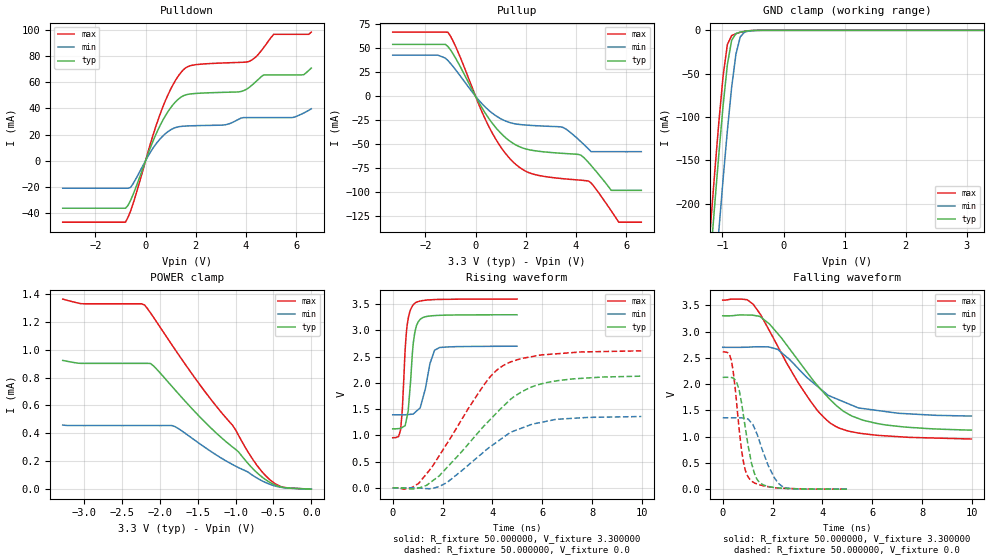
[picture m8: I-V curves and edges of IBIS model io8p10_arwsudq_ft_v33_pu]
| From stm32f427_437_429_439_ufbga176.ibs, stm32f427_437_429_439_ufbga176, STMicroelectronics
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|   Model io8p10_arwsudq_ft_v33_pu
[Model]  io8p10_arwsudq_ft_v33_pu
Model_type I/O
Polarity   Non-Inverting
Enable   Active-Low
Vinl =   0.990000V
Vinh =   2.310000V
Vmeas =  1.650000V
Cref =   40.000000pF
Rref =   100.000000M
Vref =   0.0V
C_comp   2.911600pF   2.823500pF   2.988000pF
[Temperature Range]   25.000000   0.125000k   -40.000000
[Pullup Reference]   3.300000V   2.700000V   3.600000V
[Pulldown Reference]   0.0V   0.0V   0.0V
[POWER Clamp Reference]   3.300000V   2.700000V   3.600000V
[GND Clamp Reference]   0.0V   0.0V   0.0V
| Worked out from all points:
|   slope of the pulldown table from 0 to 0.495 V, typ, clamps not added: 20.9 ohm
|   slope of the pullup table from 0 to 0.495 V, typ, clamps not added: 22.6 ohm
|   GND clamp passes 1 mA (typ) near -0.62 V on its own axis
|   rising waveform, R_fixture 50.000000, V_fixture 3.300000: 20-80 % time 219ps typ, 369ps min, 188ps max; typ from 1.12 V to 3.3 V
|   rising waveform, R_fixture 50.000000, V_fixture 0.0: 20-80 % time 2.52ns typ, 2.26ns min, 2.12ns max; typ from 0.001 V to 2.13 V
|   falling waveform, R_fixture 50.000000, V_fixture 3.300000: 20-80 % time 2.26ns typ, 2.15ns min, 2.01ns max; typ from 3.3 V to 1.12 V
|   falling waveform, R_fixture 50.000000, V_fixture 0.0: 20-80 % time 465ps typ, 673ps min, 372ps max; typ from 2.13 V to 0.001 V
[Pulldown]
|Voltage   I(typ)   I(min)   I(max)
-3.3V     -36.38mA   -21.07mA   -47.09mA
-800mV    -36.38mA   -21.07mA   -47.09mA
-600mV    -30.5mA    -20.54mA   -38.69mA
700mV     31.4mA     19.11mA    41.71mA
1.2V      45.15mA    25.37mA    61.75mA
1.6V      50.35mA    26.5mA     71.06mA
3.1V      52.28mA    27.26mA    74.76mA
4.1V      55.65mA    32.94mA    75.79mA
4.7V      65.59mA    32.94mA    86.49mA
5.1V      65.59mA    32.94mA    96.67mA
6.3V      65.82mA    36.48mA    96.67mA
6.6V      70.87mA    39.69mA    98.38mA
[Pullup]
|Voltage   I(typ)   I(min)   I(max)
-3.3V     54.07mA    42.87mA    66.93mA
-1.5V     54.07mA    42.87mA    66.93mA
-1.1V     51.86mA    37.22mA    66.7mA
500mV     -22.06mA   -14mA      -30.03mA
1.5V      -49.1mA    -28.3mA    -68.56mA
2.2V      -56.04mA   -30.32mA   -80.35mA
3.5V      -59.52mA   -32.65mA   -85.91mA
4.2V      -61.45mA   -47.47mA   -87.45mA
4.5V      -69.09mA   -55.01mA   -88.4mA
5.4V      -98mA      -57.7mA    -119.3mA
5.7V      -98mA      -57.7mA    -131.2mA
6.6V      -98mA      -57.7mA    -131.2mA
[GND_clamp]
|Voltage   I(typ)   I(min)   I(max)
-3.3V     -2.32A     -2.397A    -2.297A
-1.2V     -266.4mA   -356.3mA   -229.4mA
-1.13V    -203.6mA   -293.1mA   -166.3mA
-1.06V    -143.2mA   -231.4mA   -106.2mA
-990mV    -86.95mA   -171.8mA   -52.65mA
-920mV    -39.66mA   -115.8mA   -16.36mA
-850mV    -11.49mA   -65.84mA   -6.11mA
-780mV    -3.834mA   -27.59mA   -3.88mA
-710mV    -2.09mA    -7.753mA   -2.381mA
-640mV    -1.147mA   -2.129mA   -1.22mA
-570mV    -523.9uA   -800uA     -476.8uA
3.28V     0A         0A         0A
[POWER_clamp]
|Voltage   I(typ)   I(min)   I(max)
-3.28V    922.4uA    459.4uA    1.362mA
-3.04V    901.4uA    455.8uA    1.329mA
-2.2V     901.4uA    455.8uA    1.319mA
-2.08V    882.2uA    455.8uA    1.23mA
-1.8V     712.4uA    448.4uA    1.003mA
-1.4V     478.6uA    298uA      696.5uA
-1.04V    302.3uA    176.6uA    458.6uA
-800mV    163uA      108.7uA    236.3uA
-640mV    82.53uA    56.82uA    118.4uA
-520mV    40.35uA    29.6uA     55.89uA
-400mV    15.52uA    13.26uA    18.69uA
0V        0A         0A         0A
[Ramp]
| variable   typ   min   max
dV/dt_r  1.26919/2.51975n   0.81207/2.26254n   1.56466/2.11885n
dV/dt_f  1.28460/2.25239n   0.77760/2.14818n   1.57516/2.01379n
R_load = 50.000000
[Rising Waveform]
R_fixture= 50.000000
V_fixture= 3.300000
V_fixture_min= 2.700000
V_fixture_max= 3.600000
|time   V(typ)   V(min)   V(max)
0s        1.125V     1.393V     955.5mV
320.3ps   1.134V     1.393V     1.123V
390.4ps   1.154V     1.393V     1.531V
500.5ps   1.188V     1.393V     2.646V
620.6ps   1.466V     1.398V     3.224V
850.9ps   2.848V     1.42V      3.502V
1.101ns   3.211V     1.524V     3.561V
1.491ns   3.276V     2.365V     3.584V
1.682ns   3.284V     2.624V     3.589V
4.985ns   3.3V       2.7V       3.599V
[Rising Waveform]
R_fixture= 50.000000
V_fixture= 0.0
V_fixture_min= 0.0
V_fixture_max= 0.0
|time   V(typ)   V(min)   V(max)
0s        1.286mV    1.128mV    1.851mV
540.5ps   -7.725mV   1.049mV    -19.84mV
1.041ns   -1.906mV   -3.824mV   86.18mV
1.361ns   49.75mV    -14.64mV   270.5mV
2.182ns   390.3mV    104.1mV    849.5mV
3.784ns   1.24V      738.2mV    2.044V
4.505ns   1.587V     985.8mV    2.351V
5.165ns   1.83V      1.138V     2.466V
6.166ns   2.006V     1.269V     2.542V
9.97ns    2.129V     1.36V      2.612V
[Falling Waveform]
R_fixture= 50.000000
V_fixture= 3.300000
V_fixture_min= 2.700000
V_fixture_max= 3.600000
|time   V(typ)   V(min)   V(max)
0s        3.3V       2.7V       3.599V
981ps     3.315V     2.702V     3.606V
1.221ns   3.31V      2.708V     3.521V
1.502ns   3.283V     2.711V     3.334V
2.202ns   2.963V     2.661V     2.724V
3.524ns   2.136V     2.067V     1.674V
4.505ns   1.616V     1.732V     1.202V
5.185ns   1.392V     1.597V     1.091V
6.126ns   1.257V     1.503V     1.029V
9.97ns    1.125V     1.393V     955.5mV
[Falling Waveform]
R_fixture= 50.000000
V_fixture= 0.0
V_fixture_min= 0.0
V_fixture_max= 0.0
|time   V(typ)   V(min)   V(max)
0s        2.129V     1.36V      2.612V
340.3ps   2.126V     1.359V     2.461V
560.6ps   2.033V     1.359V     1.628V
680.7ps   1.834V     1.358V     1.044V
840.8ps   1.375V     1.351V     494mV
1.091ns   651.6mV    1.296V     188.5mV
1.451ns   144.3mV    945.4mV    88.08mV
1.832ns   52.17mV    443.2mV    48.03mV
2.362ns   19.36mV    61.86mV    20.23mV
4.985ns   1.286mV    1.128mV    1.851mV
